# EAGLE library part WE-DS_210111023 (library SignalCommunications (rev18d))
WE-DS D-SUB-Filter, Solder Pin Straight Characteristics Standard type filtered with 1000 pF High attenuation: max. ≥ 40 dB @ 180 MHz Choice of UNC 4/40 or through hole Rated voltage: 100 VDC Rated current @ 20 ºC: 5 A Withstand voltage: 250 VRMS Insulation resistance: min. 1000 MΩ Operating temperature: –55 ºC to +125 ºC Applications Filtering of interfaces External connection to -printer -sensor -display Details see: http://katalog.we-online.de/en/pbs/D-SUB-FILTER-STRAIGHT/210111023 2016 (C) Wurth Elektronik
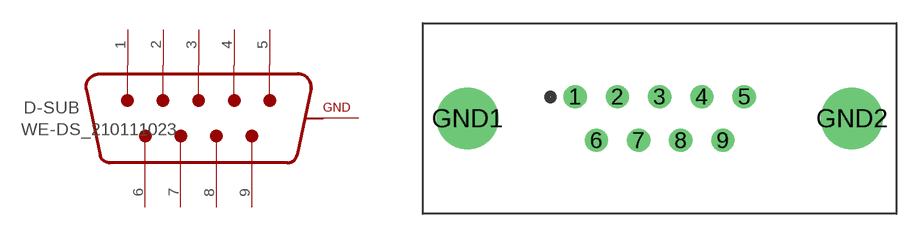
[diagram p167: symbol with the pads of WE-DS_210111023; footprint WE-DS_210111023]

Designator prefix D-SUB

## WE-DS_210111023 (WE-NUMBER: 210111023/9pins_male)  [WE-DS_210111023]
1  1  pas
2  2  pas
3  3  pas
4  4  pas
5  5  pas
6  6  pas
7  7  pas
8  8  pas
9  9  pas
GND1  GND  pwr
GND2  GND  pwr

## Footprint WE-DS_210111023 (pad centres in mm)
drill 1: 1 -5.49,1.42; 2 -2.74,1.42; 3 0,1.42; 4 2.74,1.42; 5 5.49,1.42; 6 -4.11,-1.42; 7 -1.37,-1.42; 8 1.37,-1.42; 9 4.11,-1.42
drill 3: GND1 -12.5,0; GND2 12.5,0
